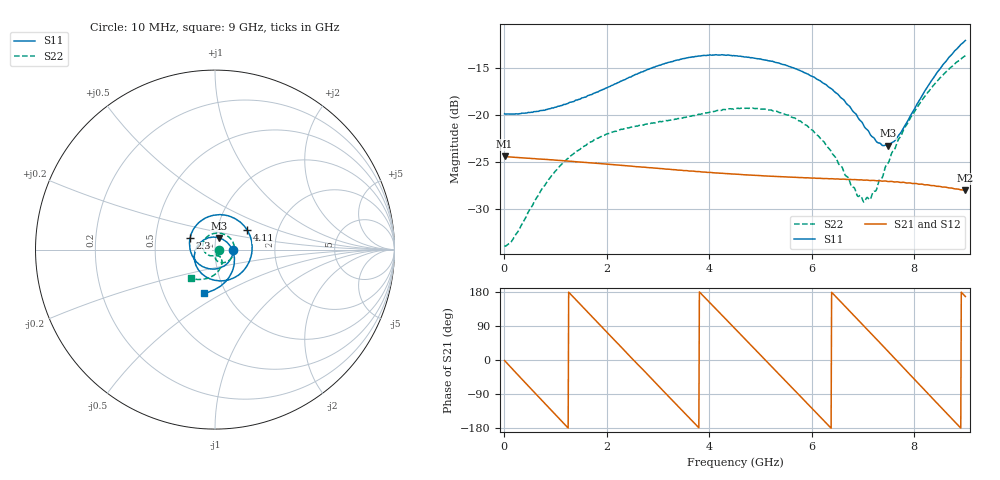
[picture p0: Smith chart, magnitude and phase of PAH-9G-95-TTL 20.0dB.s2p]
! MTS Systemtechnik GmbH
! S-Parameters
! Model: PAH-9G/95-TTL
! Attenuation Step: 20.0dB
#  HZ  S  DB  R  50.00
! Rohde & Schwarz Vector Network Analyzer
! Rohde-Schwarz,ZNB20-2Port,1334333062101652,3.45
! Created: UTC 1/26/2024, 7:20:09 AM
! freq[Hz]  db:S11  ang:S11  db:S21  ang:S21  db:S12  ang:S12  db:S22  ang:S22
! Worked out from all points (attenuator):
!   900 points, 10 MHz to 9 GHz, reference 50 ohm
!   highest |S21| = -24.36 dB at 10 MHz (marker M1); lowest = -28.0 dB at 9 GHz (marker M2)
!   lowest |S11| = -23.2 dB at 7.49 GHz (marker M3), VSWR 1.15, Z = 52 + j6.75 ohm
!   |S11| at or under -10 dB: start of sweep to end of sweep
!   |S22| runs from -34.0 to -13.6 dB; largest |S21 - S12| = 0.0016
!   S11 on the Smith chart (normalised r, x): 10 MHz: 1.23, -0.01; 2.3 GHz: 0.75, +0.10; 4.11 GHz: 1.40, +0.32; 9 GHz: 0.79, -0.41
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1e7  -19.84 -2.3  -24.36 -1.4  -24.38 -1.5  -33.88 -8.4
1.7e8  -19.86 -18.2  -24.47 -25.0  -24.48 -24.9  -33.23 -36.7
6.9e8  -19.53 -71.2  -24.66 -99.7  -24.67 -99.6  -28.30 -114.3
1.08e9  -19.03 -108.4  -24.81 -155.4  -24.82 -155.3  -25.47 -153.1
1.51e9  -18.16 -145.0  -25.00 143.4  -25.01 143.6  -23.44 171.8
1.9e9  -17.32 -175.3  -25.16 88.3  -25.18 88.3  -22.25 144.8
2.3e9  -16.33 155.6  -25.34 31.9  -25.36 31.7  -21.50 121.0
3.01e9  -14.71 106.4  -25.67 -68.1  -25.69 -68.0  -20.71 85.9
3.57e9  -13.89 67.9  -25.90 -146.7  -25.92 -146.3  -20.17 62.4
4.11e9  -13.57 31.0  -26.13 137.8  -26.15 138.3  -19.58 38.8
4.51e9  -13.66 4.0  -26.27 82.0  -26.29 82.4  -19.27 19.9
5.34e9  -14.41 -54.3  -26.53 -34.3  -26.55 -33.3  -19.62 -23.9
6.01e9  -15.85 -106.2  -26.69 -128.1  -26.70 -126.9  -21.57 -61.6
6.52e9  -17.79 -152.0  -26.79 160.3  -26.81 161.4  -25.11 -84.1
7.02e9  -21.13 151.1  -26.92 89.7  -26.91 90.9  -29.25 -75.2
7.25e9  -22.70 115.0  -26.99 57.2  -26.98 58.2  -28.06 -58.2
7.49e9  -23.24 70.0  -27.06 22.9  -27.05 24.1  -25.12 -53.0
7.51e9  -23.21 65.8  -27.06 20.2  -27.04 21.3  -24.92 -54.1
7.74e9  -21.84 24.2  -27.16 -12.9  -27.14 -11.2  -22.22 -59.9
8.24e9  -17.15 -40.8  -27.41 -84.3  -27.42 -82.9  -17.73 -85.4
8.59e9  -14.44 -72.5  -27.65 -134.2  -27.69 -132.8  -15.53 -105.7
9e9  -12.02 -104.8  -28.01 167.4  -28.08 168.9  -13.64 -129.4
